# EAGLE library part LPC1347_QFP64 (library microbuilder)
LPC1347 - ARM Cortex M3 72MHz MCU Supply: 2.0-3.6V 12-bit 500kHz ADC Flash: 64KB EEPROM: 4KB SRAM: 8KB SRAM0 + 2KB SRAM1 + 2KB USB Temp: -40°C - 85°C
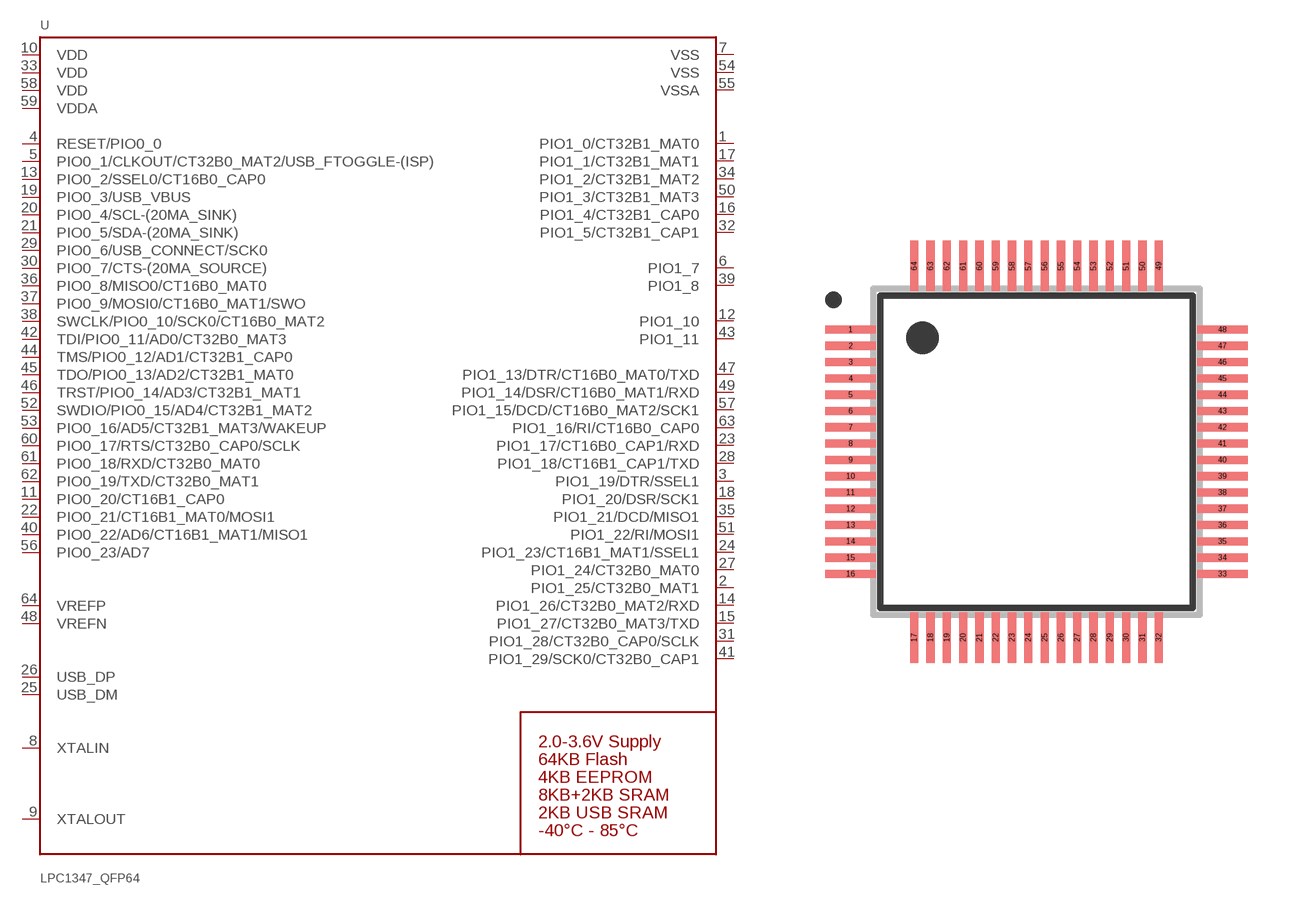
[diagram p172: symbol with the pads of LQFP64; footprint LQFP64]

Designator prefix U

## LPC1347_QFP64  [LQFP64]
1  PIO1_0/CT32B1_MAT0
2  PIO1_25/CT32B0_MAT1
3  PIO1_19/DTR/SSEL1
4  RESET/PIO0_0
5  PIO0_1/CLKOUT/CT32B0_MAT2/USB_FTOGGLE-(ISP)
6  PIO1_7
7  VSS  pwr
8  XTALIN
9  XTALOUT
10  VDD  pwr
11  PIO0_20/CT16B1_CAP0
12  PIO1_10
13  PIO0_2/SSEL0/CT16B0_CAP0
14  PIO1_26/CT32B0_MAT2/RXD
15  PIO1_27/CT32B0_MAT3/TXD
16  PIO1_4/CT32B1_CAP0
17  PIO1_1/CT32B1_MAT1
18  PIO1_20/DSR/SCK1
19  PIO0_3/USB_VBUS
20  PIO0_4/SCL-(20MA_SINK)
21  PIO0_5/SDA-(20MA_SINK)
22  PIO0_21/CT16B1_MAT0/MOSI1
23  PIO1_17/CT16B0_CAP1/RXD
24  PIO1_23/CT16B1_MAT1/SSEL1
25  USB_DM
26  USB_DP
27  PIO1_24/CT32B0_MAT0
28  PIO1_18/CT16B1_CAP1/TXD
29  PIO0_6/USB_CONNECT/SCK0
30  PIO0_7/CTS-(20MA_SOURCE)
31  PIO1_28/CT32B0_CAP0/SCLK
32  PIO1_5/CT32B1_CAP1
33  VDD  pwr
34  PIO1_2/CT32B1_MAT2
35  PIO1_21/DCD/MISO1
36  PIO0_8/MISO0/CT16B0_MAT0
37  PIO0_9/MOSI0/CT16B0_MAT1/SWO
38  SWCLK/PIO0_10/SCK0/CT16B0_MAT2
39  PIO1_8
40  PIO0_22/AD6/CT16B1_MAT1/MISO1
41  PIO1_29/SCK0/CT32B0_CAP1
42  TDI/PIO0_11/AD0/CT32B0_MAT3
43  PIO1_11
44  TMS/PIO0_12/AD1/CT32B1_CAP0
45  TDO/PIO0_13/AD2/CT32B1_MAT0
46  TRST/PIO0_14/AD3/CT32B1_MAT1
47  PIO1_13/DTR/CT16B0_MAT0/TXD
48  VREFN
49  PIO1_14/DSR/CT16B0_MAT1/RXD
50  PIO1_3/CT32B1_MAT3
51  PIO1_22/RI/MOSI1
52  SWDIO/PIO0_15/AD4/CT32B1_MAT2
53  PIO0_16/AD5/CT32B1_MAT3/WAKEUP
54  VSS  pwr
55  VSSA  pwr
56  PIO0_23/AD7
57  PIO1_15/DCD/CT16B0_MAT2/SCK1
58  VDD  pwr
59  VDDA  pwr
60  PIO0_17/RTS/CT32B0_CAP0/SCLK
61  PIO0_18/RXD/CT32B0_MAT0
62  PIO0_19/TXD/CT32B0_MAT1
63  PIO1_16/RI/CT16B0_CAP0
64  VREFP

## Footprint LQFP64 (pad centres in mm)
smd 1.55 x 0.25: 1 -5.7,3.75; 2 -5.7,3.25; 3 -5.7,2.75; 4 -5.7,2.25; 5 -5.7,1.75; 6 -5.7,1.25; 7 -5.7,0.75; 8 -5.7,0.25; 9 -5.7,-0.25; 10 -5.7,-0.75; 11 -5.7,-1.25; 12 -5.7,-1.75; 13 -5.7,-2.25; 14 -5.7,-2.75; 15 -5.7,-3.25; 16 -5.7,-3.75; 33 5.7,-3.75; 34 5.7,-3.25; 35 5.7,-2.75; 36 5.7,-2.25; 37 5.7,-1.75; 38 5.7,-1.25; 39 5.7,-0.75; 40 5.7,-0.25; 41 5.7,0.25; 42 5.7,0.75; 43 5.7,1.25; 44 5.7,1.75; 45 5.7,2.25; 46 5.7,2.75; 47 5.7,3.25; 48 5.7,3.75
smd 0.25 x 1.55: 17 -3.75,-5.7; 18 -3.25,-5.7; 19 -2.75,-5.7; 20 -2.25,-5.7; 21 -1.75,-5.7; 22 -1.25,-5.7; 23 -0.75,-5.7; 24 -0.25,-5.7; 25 0.25,-5.7; 26 0.75,-5.7; 27 1.25,-5.7; 28 1.75,-5.7; 29 2.25,-5.7; 30 2.75,-5.7; 31 3.25,-5.7; 32 3.75,-5.7; 49 3.75,5.7; 50 3.25,5.7; 51 2.75,5.7; 52 2.25,5.7; 53 1.75,5.7; 54 1.25,5.7; 55 0.75,5.7; 56 0.25,5.7; 57 -0.25,5.7; 58 -0.75,5.7; 59 -1.25,5.7; 60 -1.75,5.7; 61 -2.25,5.7; 62 -2.75,5.7; 63 -3.25,5.7; 64 -3.75,5.7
